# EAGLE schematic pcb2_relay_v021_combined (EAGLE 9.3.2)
Switching done with 23 x G6K-2F-Y 2xDPDT relays + 3 x HC-595

## Sheet 1 of 5: Voltage Controlled Bandpass Filters
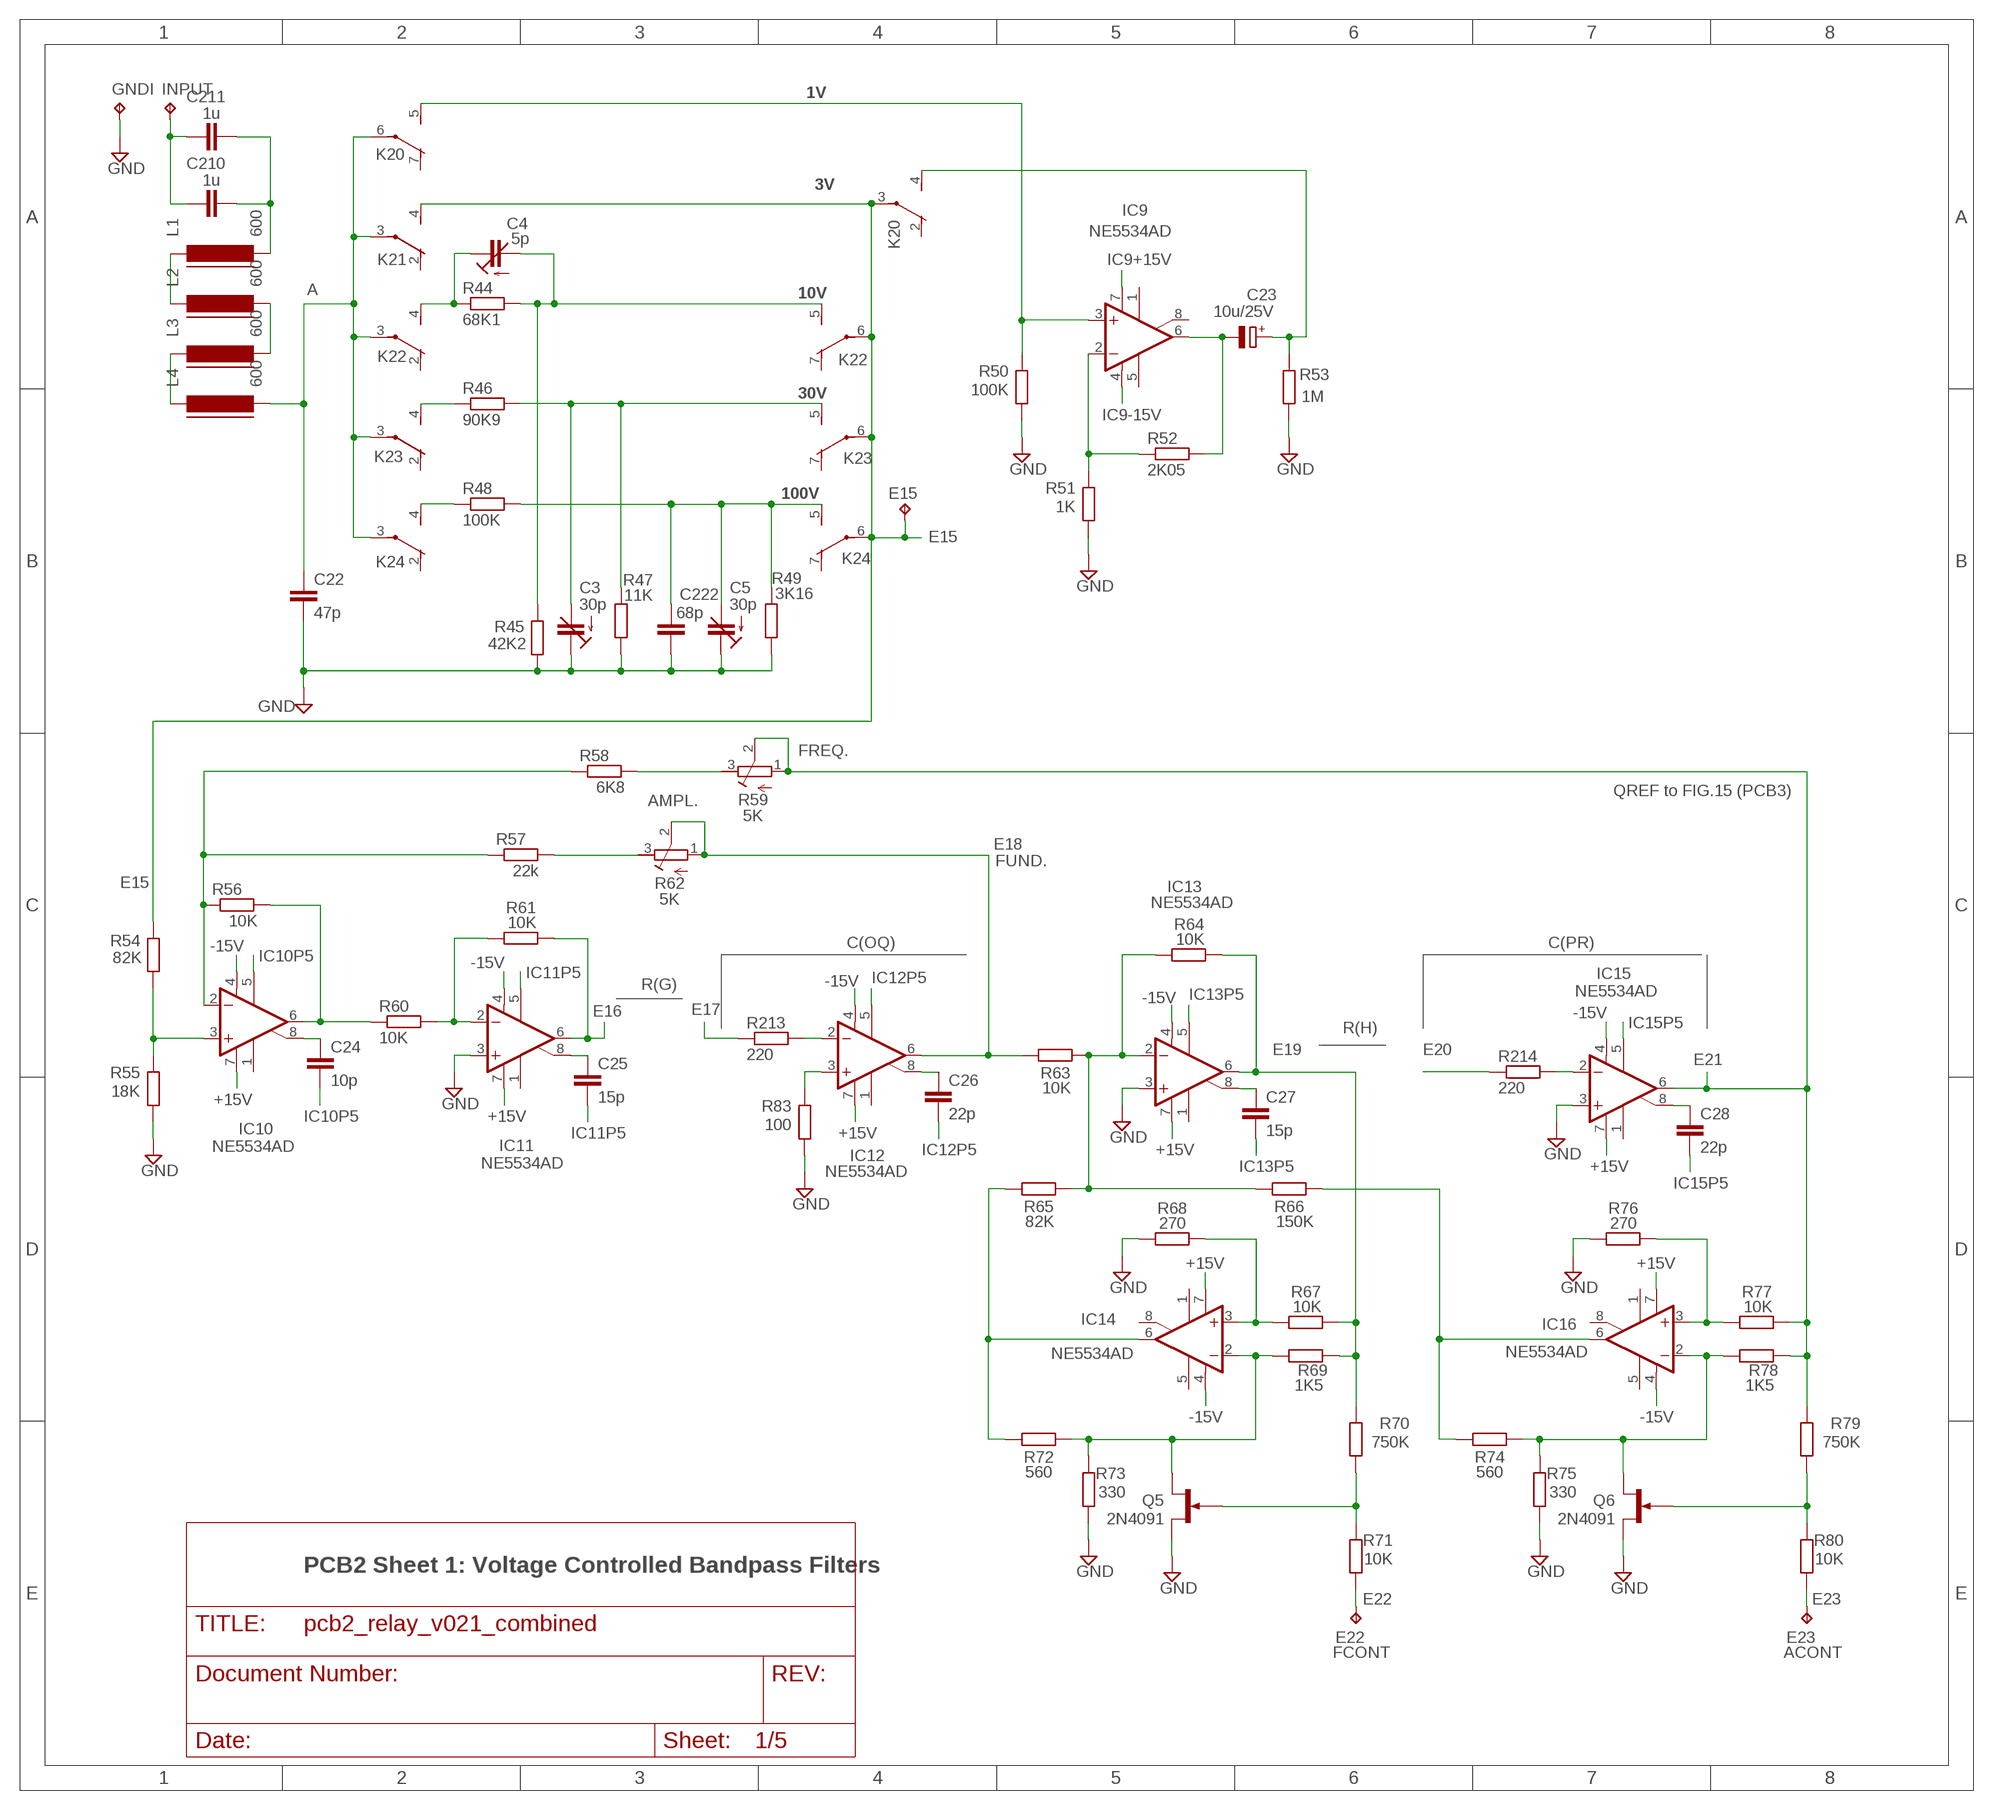
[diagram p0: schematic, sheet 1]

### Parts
C3  30p  C-TRIMM3050.504  [CTRIM3050.504]
C4  5p  C-TRIMM3050.504  [CTRIM3050.504]
C5  30p  C-TRIMM3050.504  [CTRIM3050.504]
C22  47p  C-EU075-042X103  [C075-042X103]
C23  10u/25V  CPOL-EUUD-4X5,8  [UD-4X5,8_NICHICON]
C24  10p  C-EU075-042X103  [C075-042X103]
C25  15p  C-EU075-042X103  [C075-042X103]
C26  22p  C-EU075-042X103  [C075-042X103]
C27  15p  C-EU075-042X103  [C075-042X103]
C28  22p  C-EU075-042X103  [C075-042X103]
C210  1u  C-EU150-072X183  [C150-072X183]
C211  1u  C-EU150-072X183  [C150-072X183]
C222  68p  C-EU075-052X106  [C075-052X106]
E15  TPPAD1-13Y  [P1-13Y]
E22  TPPAD1-13Y  [P1-13Y]
E23  TPPAD1-13Y  [P1-13Y]
GNDI  TPPAD1-13Y  [P1-13Y]
IC9  NE5534AD  [SO08]
IC10  NE5534AD  [SO08]
IC11  NE5534AD  [SO08]
IC12  NE5534AD  [SO08]
IC13  NE5534AD  [SO08]
IC14  NE5534AD  [SO08]
IC15  NE5534AD  [SO08]
IC16  NE5534AD  [SO08]
INPUT  TPPAD1-13Y  [P1-13Y]
K20  G6K-2F-Y  [G6K-2F-Y]
K21  G6K-2F-Y  [G6K-2F-Y]
K22  G6K-2F-Y  [G6K-2F-Y]
K23  G6K-2F-Y  [G6K-2F-Y]
K24  G6K-2F-Y  [G6K-2F-Y]
L1  600  FERRITE-1206  [FB1206]
L2  600  FERRITE-1206  [FB1206]
L3  600  FERRITE-1206  [FB1206]
L4  600  FERRITE-1206  [FB1206]
Q5  2N4091  2N5638  [TO92G]
Q6  2N4091  2N5638  [TO92G]
R44  68K1  R-EU_R1206  [R1206]
R45  42K2  R-EU_R1206  [R1206]
R46  90K9  R-EU_R1206  [R1206]
R47  11K  R-EU_R1206  [R1206]
R48  100K  R-EU_R1206  [R1206]
R49  3K16  R-EU_R1206  [R1206]
R50  100K  R-EU_R1206  [R1206]
R51  1K  R-EU_R1206  [R1206]
R52  2K05  R-EU_R1206  [R1206]
R53  1M  R-EU_R1206  [R1206]
R54  82K  R-EU_R1206  [R1206]
R55  18K  R-EU_R1206  [R1206]
R56  10K  R-EU_R1206  [R1206]
R57  22k  R-EU_R1206  [R1206]
R58  6K8  R-EU_R1206  [R1206]
R59  5K  R-TRIMM3296W  [RTRIM3296W]
R60  10K  R-EU_R1206  [R1206]
R61  10K  R-EU_R1206  [R1206]
R62  5K  R-TRIMM3296W  [RTRIM3296W]
R63  10K  R-EU_R1206  [R1206]
R64  10K  R-EU_R1206  [R1206]
R65  82K  R-EU_R1206  [R1206]
R66  150K  R-EU_R1206  [R1206]
R67  10K  R-EU_R1206  [R1206]
R68  270  R-EU_R1206  [R1206]
R69  1K5  R-EU_R1206  [R1206]
R70  750K  R-EU_R1206  [R1206]
R71  10K  R-EU_R1206  [R1206]
R72  560  R-EU_R1206  [R1206]
R73  330  R-EU_R1206  [R1206]
R74  560  R-EU_R1206  [R1206]
R75  330  R-EU_R1206  [R1206]
R76  270  R-EU_R1206  [R1206]
R77  10K  R-EU_R1206  [R1206]
R78  1K5  R-EU_R1206  [R1206]
R79  750K  R-EU_R1206  [R1206]
R80  10K  R-EU_R1206  [R1206]
R83  100  R-EU_R1206  [R1206]
R213  220  R-EU_R1206  [R1206]
R214  220  R-EU_R1206  [R1206]

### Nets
+15V: IC10.7(V+) IC11.7(V+) IC12.7(V+) IC13.7(V+) IC14.7(V+) IC15.7(V+) IC16.7(V+) ; also sheet 2,4,5
-15V: IC10.4(V-) IC11.4(V-) IC12.4(V-) IC13.4(V-) IC14.4(V-) IC15.4(V-) IC16.4(V-) ; also sheet 2,4,5
A: C22.1 K20.6(3:P) K21.3(2:P) K22.3(2:P) K23.3(2:P) K24.3(2:P) L4.2
E12: IC9.3(+IN) K20.5(3:S) R50.2
E13: C23.+ K20.4(2:S) R53.2
E15: E15.TP K20.3(2:P) K21.4(2:S) K22.6(3:P) K23.6(3:P) K24.6(3:P) R54.2 ; also sheet 2
E16: IC11.6(OUT) R61.2 ; also sheet 3
E17: R213.1 ; also sheet 3
E18: IC12.6(OUT) R62.1(A) R62.2(S) R63.2 ; also sheet 2,3,5
E19: IC13.6(OUT) R64.2 R67.2 R69.2 R70.2 ; also sheet 3
E20: R214.1 ; also sheet 3
E21: IC15.6(OUT) R59.1(A) R59.2(S) R77.2 R78.2 R79.2 ; also sheet 3
E22: E22.TP R71.1 ; also sheet 3
E23: E23.TP R80.1 ; also sheet 3
GND: C3.1(E) C5.1(E) C22.2 C222.2 GNDI.TP IC11.3(+IN) IC13.3(+IN) IC15.3(+IN) Q5.S Q6.S R45.1 R47.1 R49.1 R50.1 R51.1 R53.1 R55.1 R68.1 R73.1 R75.1 R76.1 R83.1 ; also sheet 2,3,4,5
IC9+15V: IC9.7(V+) ; also sheet 4
IC9-15V: IC9.4(V-) ; also sheet 4
IC10P5: C24.2 IC10.5(CMP)
IC11P5: C25.2 IC11.5(CMP)
IC12P5: C26.2 IC12.5(CMP)
IC13P5: C27.2 IC13.5(CMP)
IC15P5: C28.2 IC15.5(CMP)
IN: C210.1 C211.1 INPUT.TP
N$12: C24.1 IC10.8(ON/CMP)
N$26: IC10.6(OUT) R56.2 R60.1
N$27: IC11.2(-IN) R60.2 R61.1
N$31: C25.1 IC11.8(ON/CMP)
N$32: IC12.2(-IN) R213.2
N$33: C23.- IC9.6(OUT) R52.2
N$34: IC9.2(-IN) R51.2 R52.1
N$35: C26.1 IC12.8(ON/CMP)
N$38: IC10.3(+IN) R54.1 R55.2
N$39: IC12.3(+IN) R83.2
N$40: IC13.2(-IN) R63.1 R64.1 R65.1 R66.2
N$41: C27.1 IC13.8(ON/CMP)
N$42: IC14.6(OUT) R65.2 R72.2
N$43: IC14.3(+IN) R67.1 R68.2
N$44: Q5.G R70.1 R71.2
N$45: IC14.2(-IN) Q5.D R69.1 R72.1 R73.2
N$46: IC16.3(+IN) R76.2 R77.1
N$47: Q6.G R79.1 R80.2
N$48: IC16.2(-IN) Q6.D R74.1 R75.2 R78.1
N$49: IC16.6(OUT) R66.1 R74.2
N$51: C28.1 IC15.8(ON/CMP)
N$52: IC15.2(-IN) R214.2
N$53: R57.2 R62.3(E)
N$54: R58.2 R59.3(E)
N$56: IC10.2(-IN) R56.1 R57.1 R58.1
N$119: C210.2 C211.2 L1.2
N$120: C4.2(A) K22.5(3:S) R44.2 R45.2
N$121: L1.1 L2.1
N$122: L2.2 L3.2
N$123: L3.1 L4.1
N$124: C4.1(E) K22.4(2:S) R44.1
N$126: K23.4(2:S) R46.1
N$133: K24.4(2:S) R48.1
N$134: C3.2(A) K23.5(3:S) R46.2 R47.2
N$137: C5.2(A) C222.1 K24.5(3:S) R48.2 R49.2
Unconnected: IC9.1(ON) IC9.5(CMP) IC9.8(ON/CMP) IC10.1(ON) IC11.1(ON) IC12.1(ON) IC13.1(ON) IC14.1(ON) IC14.5(CMP) IC14.8(ON/CMP) IC15.1(ON) IC16.1(ON) IC16.5(CMP) IC16.8(ON/CMP) K20.2(2:O) K20.7(3:O) K21.2(2:O) K22.2(2:O) K22.7(3:O) K23.2(2:O) K23.7(3:O) K24.2(2:O) K24.7(3:O)

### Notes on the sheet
- 1V
- 3V
- 10V
- 30V
- 100V
- FREQ.
- QREF to FIG.15 (PCB3)
- AMPL.
- FUND.
- C(OQ) | C(PR)
- R(G)
- R(H)
- PCB2 Sheet 1: Voltage Controlled Bandpass Filters
- FCONT | ACONT

## Sheet 2 of 5: Product Amplifier and Level Set
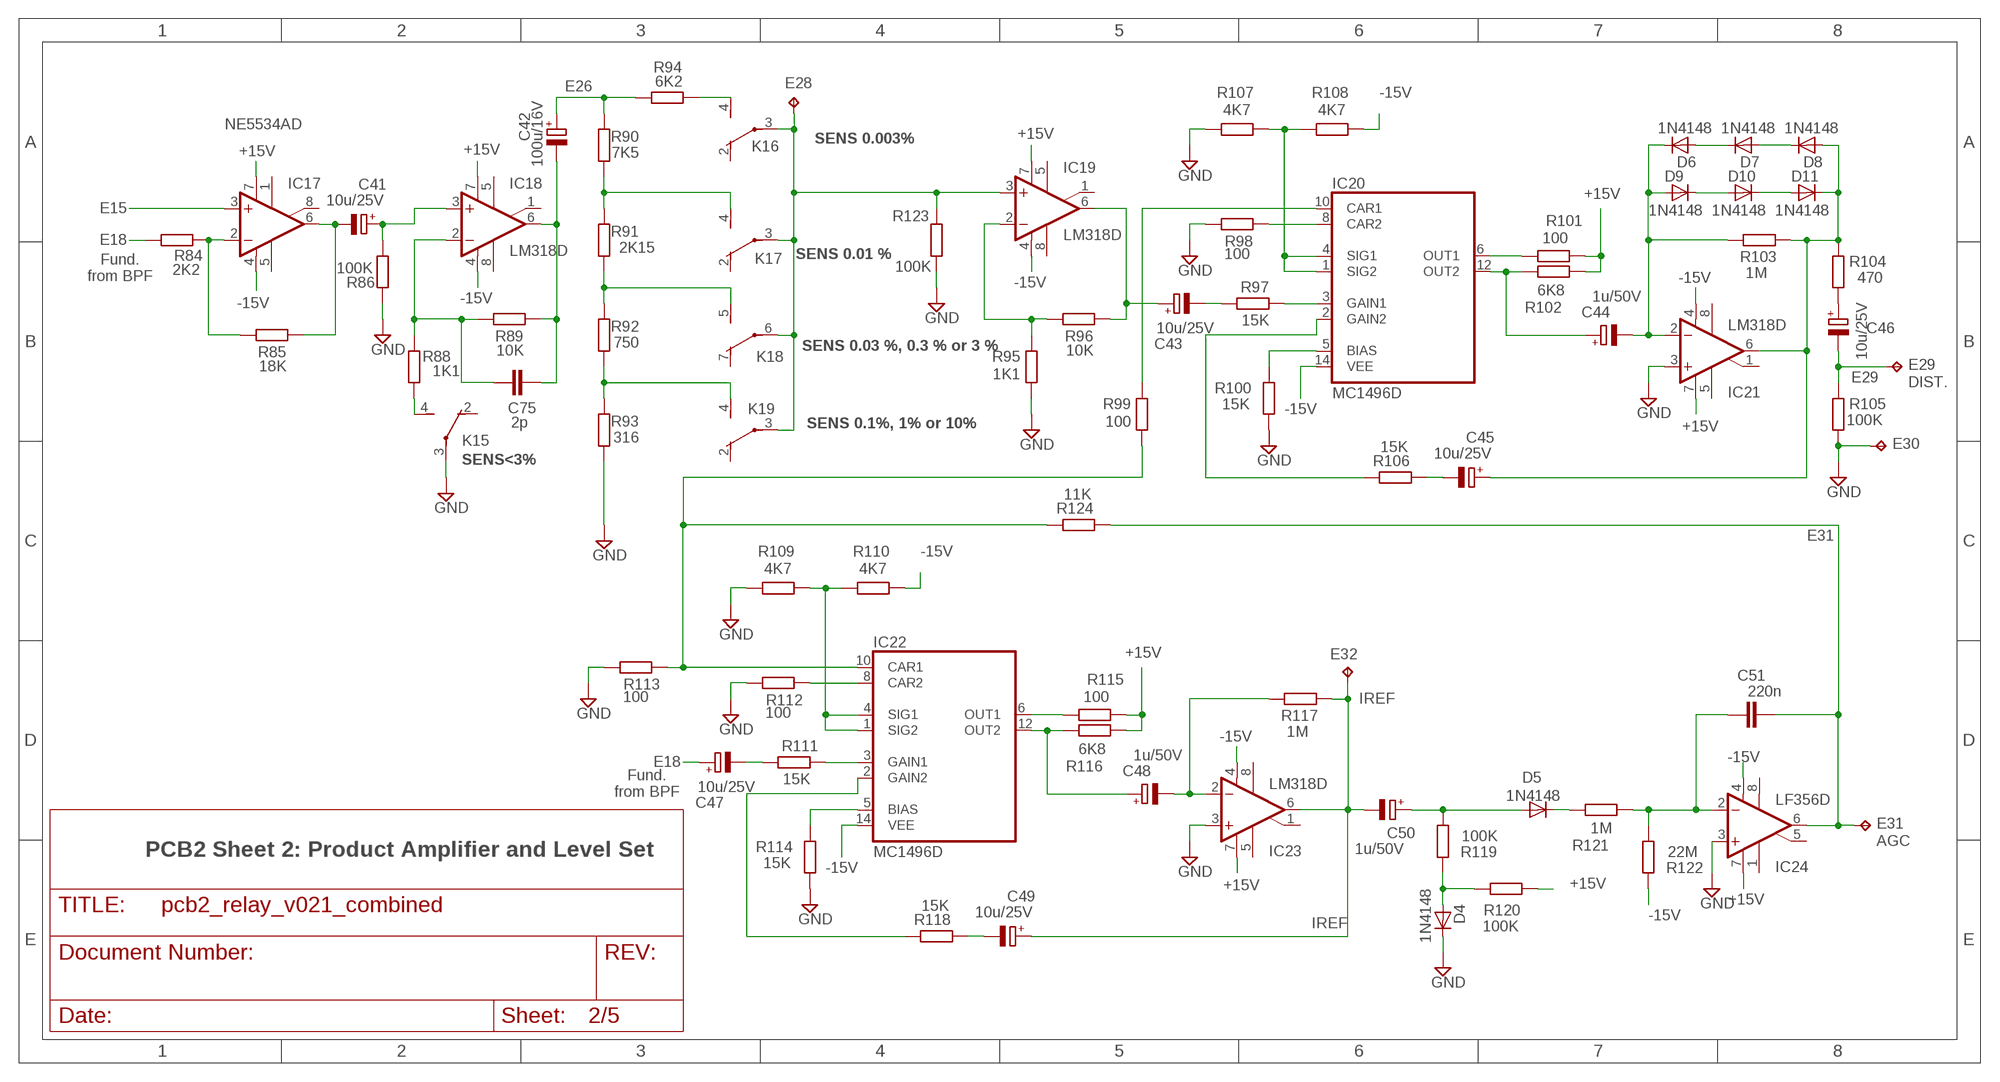
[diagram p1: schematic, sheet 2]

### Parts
C41  10u/25V  CPOL-EUUD-4X5,8  [UD-4X5,8_NICHICON]
C42  100u/16V  CPOL-EUUD-6,3X8,8  [UD-6,3X5,8_NICHICON]
C43  10u/25V  CPOL-EUUD-4X5,8  [UD-4X5,8_NICHICON]
C44  1u/50V  CPOL-EUUD-4X5,8  [UD-4X5,8_NICHICON]
C45  10u/25V  CPOL-EUUD-4X5,8  [UD-4X5,8_NICHICON]
C46  10u/25V  CPOL-EUUD-4X5,8  [UD-4X5,8_NICHICON]
C47  10u/25V  CPOL-EUUD-4X5,8  [UD-4X5,8_NICHICON]
C48  1u/50V  CPOL-EUUD-4X5,8  [UD-4X5,8_NICHICON]
C49  10u/25V  CPOL-EUUD-4X5,8  [UD-4X5,8_NICHICON]
C50  1u/50V  CPOL-EUUD-4X5,8  [UD-4X5,8_NICHICON]
C51  220n  C-EU075-052X106  [C075-052X106]
C75  2p  C-EUC1206  [C1206]
D4  1N4148  D-SOD-80  [SOD80]
D5  1N4148  D-SOD-80  [SOD80]
D6  1N4148  D-SOD-80  [SOD80]
D7  1N4148  D-SOD-80  [SOD80]
D8  1N4148  D-SOD-80  [SOD80]
D9  1N4148  D-SOD-80  [SOD80]
D10  1N4148  D-SOD-80  [SOD80]
D11  1N4148  D-SOD-80  [SOD80]
E28  TPPAD1-13Y  [P1-13Y]
E29  TPPAD1-13Y  [P1-13Y]
E30  TPPAD1-13Y  [P1-13Y]
E31  TPPAD1-13Y  [P1-13Y]
E32  TPPAD1-13Y  [P1-13Y]
IC17  NE5534AD  [SO08]
IC18  LM318D  [SO08]
IC19  LM318D  [SO08]
IC20  MC1496D  [SOIC-14]
IC21  LM318D  [SO08]
IC22  MC1496D  [SOIC-14]
IC23  LM318D  [SO08]
IC24  LF356D  [SO08]
K15  G6K-2F-Y  [G6K-2F-Y]
K16  G6K-2F-Y  [G6K-2F-Y]
K17  G6K-2F-Y  [G6K-2F-Y]
K18  G6K-2F-Y  [G6K-2F-Y]
K19  G6K-2F-Y  [G6K-2F-Y]
R84  2K2  R-EU_R1206  [R1206]
R85  18K  R-EU_R1206  [R1206]
R86  100K  R-EU_R1206  [R1206]
R88  1K1  R-EU_R1206  [R1206]
R89  10K  R-EU_R1206  [R1206]
R90  7K5  R-EU_R1206  [R1206]
R91  2K15  R-EU_R1206  [R1206]
R92  750  R-EU_R1206  [R1206]
R93  316  R-EU_R1206  [R1206]
R94  6K2  R-EU_R1206  [R1206]
R95  1K1  R-EU_R1206  [R1206]
R96  10K  R-EU_R1206  [R1206]
R97  15K  R-EU_R1206  [R1206]
R98  100  R-EU_R1206  [R1206]
R99  100  R-EU_R1206  [R1206]
R100  15K  R-EU_R1206  [R1206]
R101  100  R-EU_R1206  [R1206]
R102  6K8  R-EU_R1206  [R1206]
R103  1M  R-EU_R1206  [R1206]
R104  470  R-EU_R1206  [R1206]
R105  100K  R-EU_R1206  [R1206]
R106  15K  R-EU_R1206  [R1206]
R107  4K7  R-EU_R1206  [R1206]
R108  4K7  R-EU_R1206  [R1206]
R109  4K7  R-EU_R1206  [R1206]
R110  4K7  R-EU_R1206  [R1206]
R111  15K  R-EU_R1206  [R1206]
R112  100  R-EU_R1206  [R1206]
R113  100  R-EU_R1206  [R1206]
R114  15K  R-EU_R1206  [R1206]
R115  100  R-EU_R1206  [R1206]
R116  6K8  R-EU_R1206  [R1206]
R117  1M  R-EU_R1206  [R1206]
R118  15K  R-EU_R1206  [R1206]
R119  100K  R-EU_R1206  [R1206]
R120  100K  R-EU_R1206  [R1206]
R121  1M  R-EU_R1206  [R1206]
R122  22M  R-EU_R1206  [R1206]
R123  100K  R-EU_R1206  [R1206]
R124  11K  R-EU_R1206  [R1206]

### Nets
+15V: IC17.7(V+) IC18.7(V+) IC19.7(V+) IC21.7(V+) IC23.7(V+) IC24.7(V+) R101.1 R102.2 R115.1 R116.2 R120.1 ; also sheet 1,4,5
-15V: IC17.4(V-) IC18.4(V-) IC19.4(V-) IC20.14(VEE) IC21.4(V-) IC22.14(VEE) IC23.4(V-) IC24.4(V-) R108.2 R110.2 R122.1 ; also sheet 1,4,5
E15: IC17.3(+IN) ; also sheet 1
E18: C47.+ R84.2 ; also sheet 1,3,5
E25: K15.4(2:S) R88.2
E26: C42.+ R90.1 R94.2
E28: E28.TP IC19.3(+IN) K16.3(2:P) K17.3(2:P) K18.6(3:P) K19.3(2:P) R123.2
E29: C46.- E29.TP R105.1 ; also sheet 3
E31: C51.2 E31.TP IC24.6(OUT) R124.2 ; also sheet 3
GND: D4.1(C) E30.TP IC21.3(+IN) IC23.3(+IN) IC24.3(+IN) K15.3(2:P) R86.1 R93.2 R95.2 R98.2 R100.2 R105.2 R107.1 R109.1 R112.2 R113.2 R114.2 R123.1 ; also sheet 1,3,4,5
IREF: C49.+ C50.- E32.TP IC23.6(OUT) R117.2 ; also sheet 3
N$3: K19.4(2:S) R92.2 R93.1
N$4: K18.5(3:S) R91.2 R92.1
N$5: K17.4(2:S) R90.2 R91.1
N$6: K16.4(2:S) R94.1
N$17: IC17.2(-IN) R84.1 R85.2
N$22: C41.- IC17.6(OUT) R85.1
N$24: C41.+ IC18.3(+IN) R86.2
N$28: C75.2 IC18.2(-IN) R88.1 R89.2
N$29: C42.- C75.1 IC18.6(OUT) R89.1
N$36: IC19.2(-IN) R95.1 R96.2
N$37: C43.+ IC19.6(OUT) R96.1
N$57: C43.- R97.2
N$58: IC20.3(GAIN1) R97.1
N$59: IC20.5(BIAS) R100.1
N$60: IC20.2(GAIN2) R106.1
N$61: C45.- R106.2
N$62: IC20.1(SIG2) IC20.4(SIG1) R107.2 R108.1
N$64: IC20.8(CAR2) R98.1
N$65: IC20.10(CAR1) R99.1
N$66: IC20.6(OUT1) R101.2
N$67: C44.+ IC20.12(OUT2) R102.1
N$68: C45.+ D8.2(A) D11.1(C) IC21.6(OUT) R103.2 R104.1
N$69: C44.- D6.1(C) D9.2(A) IC21.2(-IN) R103.1
N$70: D9.1(C) D10.2(A)
N$125: D10.1(C) D11.2(A)
N$135: D7.2(A) D8.1(C)
N$136: D6.2(A) D7.1(C)
N$138: C46.+ R104.2
N$139: C47.- R111.2
N$157: IC22.3(GAIN1) R111.1
N$158: IC22.5(BIAS) R114.1
N$159: IC22.2(GAIN2) R118.1
N$160: C49.- R118.2
N$161: IC22.1(SIG2) IC22.4(SIG1) R109.2 R110.1
N$162: IC22.8(CAR2) R112.1
N$163: IC22.6(OUT1) R115.2
N$164: C48.+ IC22.12(OUT2) R116.1
N$165: C48.- IC23.2(-IN) R117.1
N$166: IC22.10(CAR1) R99.2 R113.1 R124.1
N$167: C51.1 IC24.2(-IN) R121.2 R122.2
N$168: D5.1(C) R121.1
N$169: D4.2(A) R119.1 R120.2
N$170: C50.+ D5.2(A) R119.2
Unconnected: IC17.1(ON) IC17.5(CMP) IC17.8(ON/CMP) IC18.1(ON/CMP) IC18.5(ON) IC18.8(CMP) IC19.1(ON/CMP) IC19.5(ON) IC19.8(CMP) IC21.1(ON/CMP) IC21.5(ON) IC21.8(CMP) IC23.1(ON/CMP) IC23.5(ON) IC23.8(CMP) IC24.1(ON1) IC24.5(ON2) IC24.8(OPT) K15.2(2:O) K16.2(2:O) K17.2(2:O) K18.7(3:O) K19.2(2:O)

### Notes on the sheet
- SENS 0.003%
- SENS 0.01 %
- Fund.
  from BPF
- SENS 0.03 %, 0.3 % or 3 %
- DIST.
- SENS 0.1%, 1% or 10%
- SENS<3%
- IREF
- Fund.
  from BPF
- AGC
- PCB2 Sheet 2: Product Amplifier and Level Set

## Sheet 3 of 5: Relays + Digital Logic
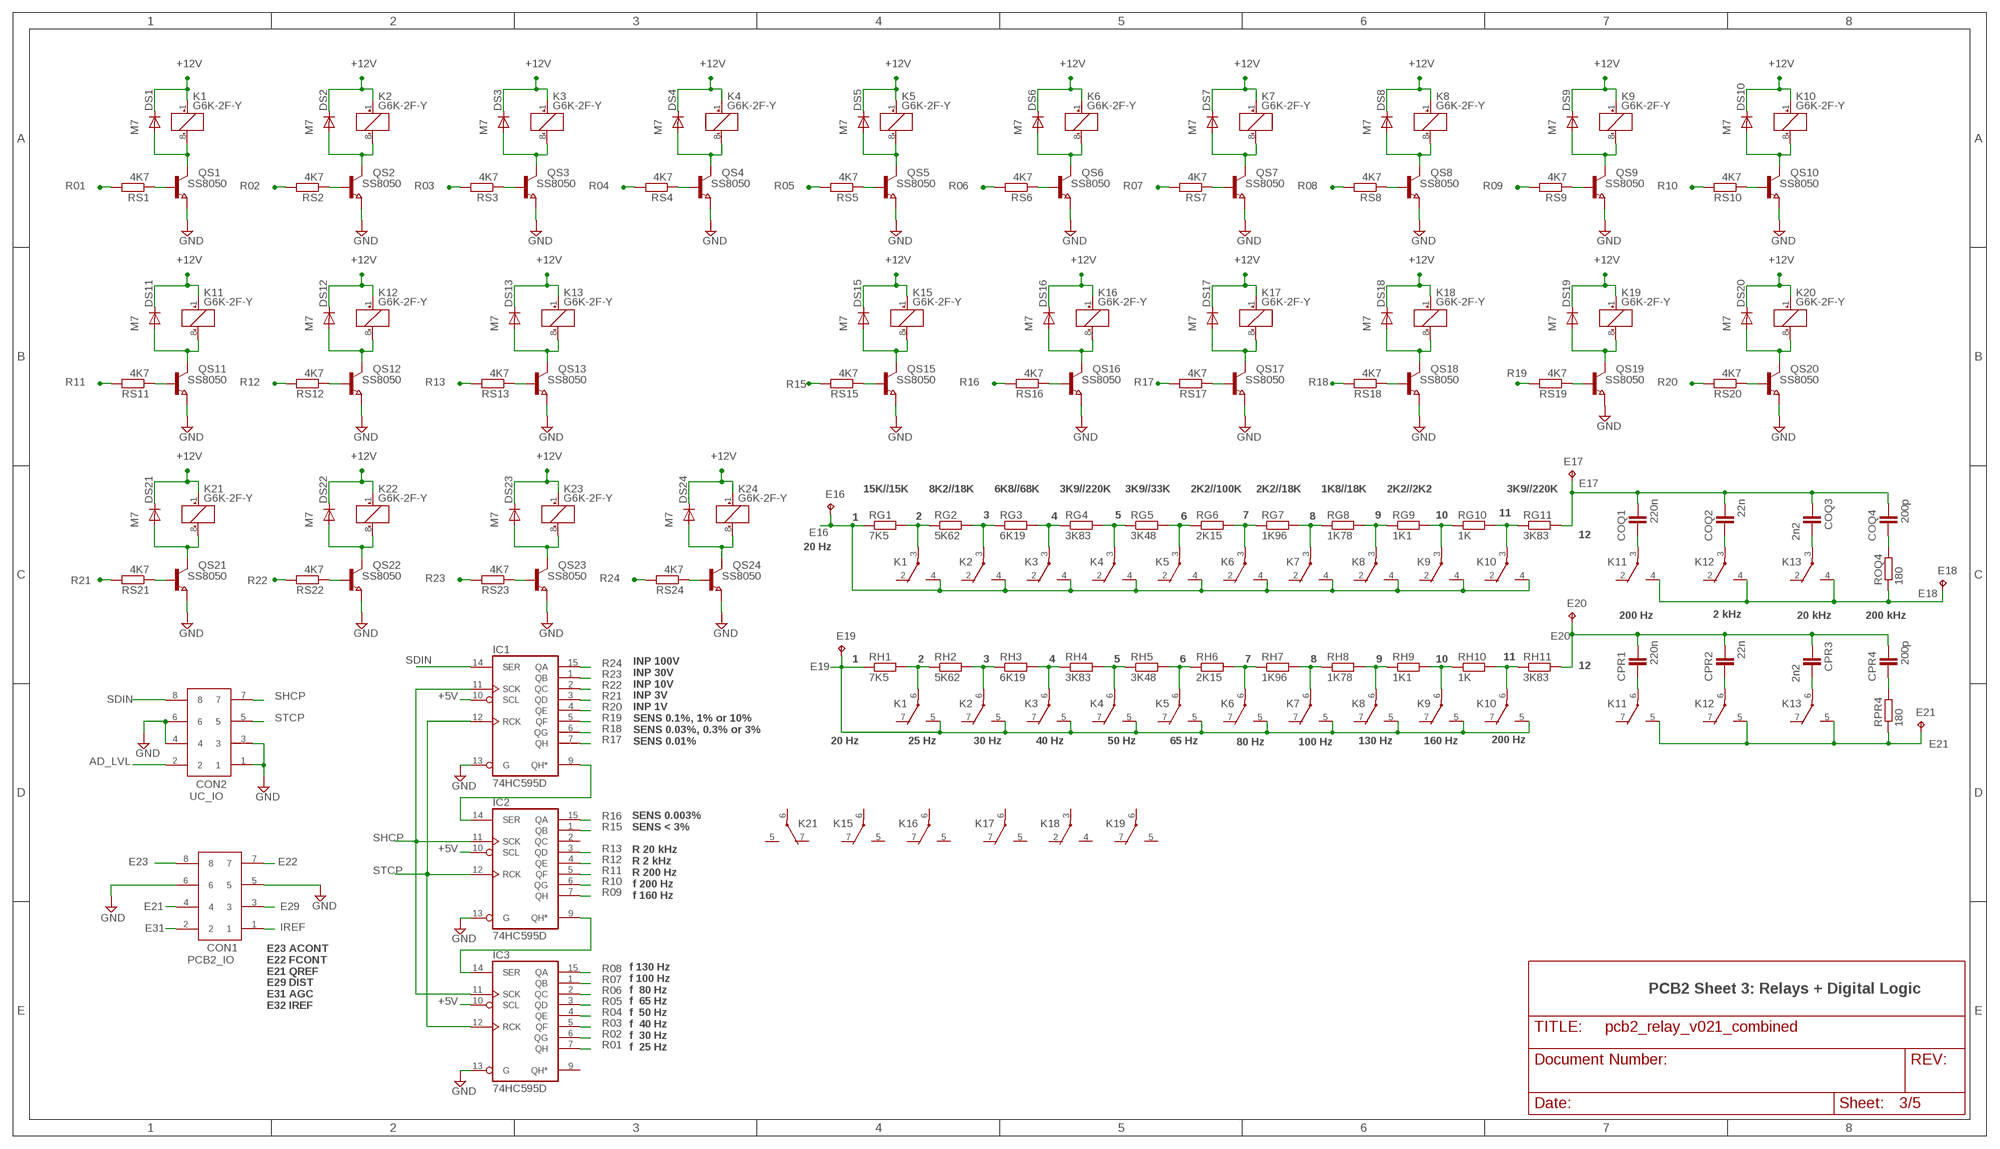
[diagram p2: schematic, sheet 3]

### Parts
CON1  PCB2_IO  61200821621  [61200821621]
CON2  UC_IO  61200821621  [61200821621]
COQ1  220n  C-EU075-052X106  [C075-052X106]
COQ2  22n  C-EU050-045X075  [C050-045X075]
COQ3  2n2  C-EU075-052X106  [C075-052X106]
COQ4  200p  C-EU102-043X133  [C102-043X133]
CPR1  220n  C-EU075-052X106  [C075-052X106]
CPR2  22n  C-EU050-045X075  [C050-045X075]
CPR3  2n2  C-EU075-052X106  [C075-052X106]
CPR4  200p  C-EU102-043X133  [C102-043X133]
DS1  M7  DIODE-DO214AC  [DO214AC]
DS2  M7  DIODE-DO214AC  [DO214AC]
DS3  M7  DIODE-DO214AC  [DO214AC]
DS4  M7  DIODE-DO214AC  [DO214AC]
DS5  M7  DIODE-DO214AC  [DO214AC]
DS6  M7  DIODE-DO214AC  [DO214AC]
DS7  M7  DIODE-DO214AC  [DO214AC]
DS8  M7  DIODE-DO214AC  [DO214AC]
DS9  M7  DIODE-DO214AC  [DO214AC]
DS10  M7  DIODE-DO214AC  [DO214AC]
DS11  M7  DIODE-DO214AC  [DO214AC]
DS12  M7  DIODE-DO214AC  [DO214AC]
DS13  M7  DIODE-DO214AC  [DO214AC]
DS15  M7  DIODE-DO214AC  [DO214AC]
DS16  M7  DIODE-DO214AC  [DO214AC]
DS17  M7  DIODE-DO214AC  [DO214AC]
DS18  M7  DIODE-DO214AC  [DO214AC]
DS19  M7  DIODE-DO214AC  [DO214AC]
DS20  M7  DIODE-DO214AC  [DO214AC]
DS21  M7  DIODE-DO214AC  [DO214AC]
DS22  M7  DIODE-DO214AC  [DO214AC]
DS23  M7  DIODE-DO214AC  [DO214AC]
DS24  M7  DIODE-DO214AC  [DO214AC]
E16  TPPAD1-13Y  [P1-13Y]
E17  TPPAD1-13Y  [P1-13Y]
E18  TPPAD1-13Y  [P1-13Y]
E19  TPPAD1-13Y  [P1-13Y]
E20  TPPAD1-13Y  [P1-13Y]
E21  TPPAD1-13Y  [P1-13Y]
IC1  74HC595D  [SO16]
IC2  74HC595D  [SO16]
IC3  74HC595D  [SO16]
K1  G6K-2F-Y  [G6K-2F-Y]
K2  G6K-2F-Y  [G6K-2F-Y]
K3  G6K-2F-Y  [G6K-2F-Y]
K4  G6K-2F-Y  [G6K-2F-Y]
K5  G6K-2F-Y  [G6K-2F-Y]
K6  G6K-2F-Y  [G6K-2F-Y]
K7  G6K-2F-Y  [G6K-2F-Y]
K8  G6K-2F-Y  [G6K-2F-Y]
K9  G6K-2F-Y  [G6K-2F-Y]
K10  G6K-2F-Y  [G6K-2F-Y]
K11  G6K-2F-Y  [G6K-2F-Y]
K12  G6K-2F-Y  [G6K-2F-Y]
K13  G6K-2F-Y  [G6K-2F-Y]
QS1  SS8050  NPN-TRANSISTOR_SOT23  [SOT23]
QS2  SS8050  NPN-TRANSISTOR_SOT23  [SOT23]
QS3  SS8050  NPN-TRANSISTOR_SOT23  [SOT23]
QS4  SS8050  NPN-TRANSISTOR_SOT23  [SOT23]
QS5  SS8050  NPN-TRANSISTOR_SOT23  [SOT23]
QS6  SS8050  NPN-TRANSISTOR_SOT23  [SOT23]
QS7  SS8050  NPN-TRANSISTOR_SOT23  [SOT23]
QS8  SS8050  NPN-TRANSISTOR_SOT23  [SOT23]
QS9  SS8050  NPN-TRANSISTOR_SOT23  [SOT23]
QS10  SS8050  NPN-TRANSISTOR_SOT23  [SOT23]
QS11  SS8050  NPN-TRANSISTOR_SOT23  [SOT23]
QS12  SS8050  NPN-TRANSISTOR_SOT23  [SOT23]
QS13  SS8050  NPN-TRANSISTOR_SOT23  [SOT23]
QS15  SS8050  NPN-TRANSISTOR_SOT23  [SOT23]
QS16  SS8050  NPN-TRANSISTOR_SOT23  [SOT23]
QS17  SS8050  NPN-TRANSISTOR_SOT23  [SOT23]
QS18  SS8050  NPN-TRANSISTOR_SOT23  [SOT23]
QS19  SS8050  NPN-TRANSISTOR_SOT23  [SOT23]
QS20  SS8050  NPN-TRANSISTOR_SOT23  [SOT23]
QS21  SS8050  NPN-TRANSISTOR_SOT23  [SOT23]
QS22  SS8050  NPN-TRANSISTOR_SOT23  [SOT23]
QS23  SS8050  NPN-TRANSISTOR_SOT23  [SOT23]
QS24  SS8050  NPN-TRANSISTOR_SOT23  [SOT23]
RG1  7K5  R-EU_R1206  [R1206]
RG2  5K62  R-EU_R1206  [R1206]
RG3  6K19  R-EU_R1206  [R1206]
RG4  3K83  R-EU_R1206  [R1206]
RG5  3K48  R-EU_R1206  [R1206]
RG6  2K15  R-EU_R1206  [R1206]
RG7  1K96  R-EU_R1206  [R1206]
RG8  1K78  R-EU_R1206  [R1206]
RG9  1K1  R-EU_R1206  [R1206]
RG10  1K  R-EU_R1206  [R1206]
RG11  3K83  R-EU_R1206  [R1206]
RH1  7K5  R-EU_R1206  [R1206]
RH2  5K62  R-EU_R1206  [R1206]
RH3  6K19  R-EU_R1206  [R1206]
RH4  3K83  R-EU_R1206  [R1206]
RH5  3K48  R-EU_R1206  [R1206]
RH6  2K15  R-EU_R1206  [R1206]
RH7  1K96  R-EU_R1206  [R1206]
RH8  1K78  R-EU_R1206  [R1206]
RH9  1K1  R-EU_R1206  [R1206]
RH10  1K  R-EU_R1206  [R1206]
RH11  3K83  R-EU_R1206  [R1206]
ROQ4  180  R-EU_R1206  [R1206]
RPR4  180  R-EU_R1206  [R1206]
RS1  4K7  R-EU_R1206  [R1206]
RS2  4K7  R-EU_R1206  [R1206]
RS3  4K7  R-EU_R1206  [R1206]
RS4  4K7  R-EU_R1206  [R1206]
RS5  4K7  R-EU_R1206  [R1206]
RS6  4K7  R-EU_R1206  [R1206]
RS7  4K7  R-EU_R1206  [R1206]
RS8  4K7  R-EU_R1206  [R1206]
RS9  4K7  R-EU_R1206  [R1206]
RS10  4K7  R-EU_R1206  [R1206]
RS11  4K7  R-EU_R1206  [R1206]
RS12  4K7  R-EU_R1206  [R1206]
RS13  4K7  R-EU_R1206  [R1206]
RS15  4K7  R-EU_R1206  [R1206]
RS16  4K7  R-EU_R1206  [R1206]
RS17  4K7  R-EU_R1206  [R1206]
RS18  4K7  R-EU_R1206  [R1206]
RS19  4K7  R-EU_R1206  [R1206]
RS20  4K7  R-EU_R1206  [R1206]
RS21  4K7  R-EU_R1206  [R1206]
RS22  4K7  R-EU_R1206  [R1206]
RS23  4K7  R-EU_R1206  [R1206]
RS24  4K7  R-EU_R1206  [R1206]

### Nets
+5V: IC1.10(SCL) IC2.10(SCL) IC3.10(SCL) ; also sheet 4
+12V: DS1.C DS2.C DS3.C DS4.C DS5.C DS6.C DS7.C DS8.C DS9.C DS10.C DS11.C DS12.C DS13.C DS15.C DS16.C DS17.C DS18.C DS19.C DS20.C DS21.C DS22.C DS23.C DS24.C K1.1(1:+) K2.1(1:+) K3.1(1:+) K4.1(1:+) K5.1(1:+) K6.1(1:+) K7.1(1:+) K8.1(1:+) K9.1(1:+) K10.1(1:+) K11.1(1:+) K12.1(1:+) K13.1(1:+) K15.1(1:+) K16.1(1:+) K17.1(1:+) K18.1(1:+) K19.1(1:+) K20.1(1:+) K21.1(1:+) K22.1(1:+) K23.1(1:+) K24.1(1:+) ; also sheet 4
AD_LVL: CON2.2 ; also sheet 5
E16: E16.TP K1.4(2:S) K2.4(2:S) K3.4(2:S) K4.4(2:S) K5.4(2:S) K6.4(2:S) K7.4(2:S) K8.4(2:S) K9.4(2:S) K10.4(2:S) RG1.1 ; also sheet 1
E17: COQ1.2 COQ2.2 COQ3.1 COQ4.2 E17.TP RG11.2 ; also sheet 1
E18: E18.TP K11.4(2:S) K12.4(2:S) K13.4(2:S) ROQ4.1 ; also sheet 1,2,5
E19: E19.TP K1.5(3:S) K2.5(3:S) K3.5(3:S) K4.5(3:S) K5.5(3:S) K6.5(3:S) K7.5(3:S) K8.5(3:S) K9.5(3:S) K10.5(3:S) RH1.1 ; also sheet 1
E20: CPR1.2 CPR2.2 CPR3.1 CPR4.2 E20.TP RH11.2 ; also sheet 1
E21: CON1.4 E21.TP K11.5(3:S) K12.5(3:S) K13.5(3:S) RPR4.1 ; also sheet 1
E22: CON1.7 ; also sheet 1
E23: CON1.8 ; also sheet 1
E29: CON1.3 ; also sheet 2
E31: CON1.2 ; also sheet 2
GND: CON1.5 CON1.6 CON2.1 CON2.3 CON2.4 CON2.6 IC1.13(G) IC2.13(G) IC3.13(G) QS1.2(E) QS2.2(E) QS3.2(E) QS4.2(E) QS5.2(E) QS6.2(E) QS7.2(E) QS8.2(E) QS9.2(E) QS10.2(E) QS11.2(E) QS12.2(E) QS13.2(E) QS15.2(E) QS16.2(E) QS17.2(E) QS18.2(E) QS19.2(E) QS20.2(E) QS21.2(E) QS22.2(E) QS23.2(E) QS24.2(E) ; also sheet 1,2,4,5
IREF: CON1.1 ; also sheet 2
N$7: QS19.1(B) RS19.1
N$8: DS19.A K19.8(1:-) QS19.3(C)
N$30: K1.3(2:P) RG1.2 RG2.1
N$55: K2.3(2:P) RG2.2 RG3.1
N$63: K3.3(2:P) RG3.2 RG4.1
N$71: K4.3(2:P) RG4.2 RG5.1
N$72: K5.3(2:P) RG5.2 RG6.1
N$73: K6.3(2:P) RG6.2 RG7.1
N$74: K7.3(2:P) RG7.2 RG8.1
N$75: K8.3(2:P) RG8.2 RG9.1
N$76: K9.3(2:P) RG9.2 RG10.1
N$77: K10.3(2:P) RG10.2 RG11.1
N$78: K1.6(3:P) RH1.2 RH2.1
N$79: K2.6(3:P) RH2.2 RH3.1
N$80: K3.6(3:P) RH3.2 RH4.1
N$81: K4.6(3:P) RH4.2 RH5.1
N$82: K5.6(3:P) RH5.2 RH6.1
N$83: K6.6(3:P) RH6.2 RH7.1
N$84: K7.6(3:P) RH7.2 RH8.1
N$85: K8.6(3:P) RH8.2 RH9.1
N$86: K9.6(3:P) RH9.2 RH10.1
N$87: K10.6(3:P) RH10.2 RH11.1
N$88: QS1.1(B) RS1.1
N$89: DS1.A K1.8(1:-) QS1.3(C)
N$90: QS2.1(B) RS2.1
N$91: DS2.A K2.8(1:-) QS2.3(C)
N$92: QS3.1(B) RS3.1
N$93: DS3.A K3.8(1:-) QS3.3(C)
N$94: QS4.1(B) RS4.1
N$95: DS4.A K4.8(1:-) QS4.3(C)
N$96: QS5.1(B) RS5.1
N$97: DS5.A K5.8(1:-) QS5.3(C)
N$98: QS6.1(B) RS6.1
N$99: DS6.A K6.8(1:-) QS6.3(C)
N$100: QS7.1(B) RS7.1
N$101: DS7.A K7.8(1:-) QS7.3(C)
N$102: QS8.1(B) RS8.1
N$103: DS8.A K8.8(1:-) QS8.3(C)
N$104: QS9.1(B) RS9.1
N$105: DS9.A K9.8(1:-) QS9.3(C)
N$106: QS10.1(B) RS10.1
N$107: DS10.A K10.8(1:-) QS10.3(C)
N$108: COQ1.1 K11.3(2:P)
N$109: COQ2.1 K12.3(2:P)
N$110: COQ3.2 K13.3(2:P)
N$111: QS11.1(B) RS11.1
N$112: DS11.A K11.8(1:-) QS11.3(C)
N$113: QS12.1(B) RS12.1
N$114: DS12.A K12.8(1:-) QS12.3(C)
N$115: QS13.1(B) RS13.1
N$116: DS13.A K13.8(1:-) QS13.3(C)
N$117: QS20.1(B) RS20.1
N$118: DS20.A K20.8(1:-) QS20.3(C)
N$127: QS22.1(B) RS22.1
N$128: DS22.A K22.8(1:-) QS22.3(C)
N$129: QS23.1(B) RS23.1
N$130: DS23.A K23.8(1:-) QS23.3(C)
N$131: QS24.1(B) RS24.1
N$132: DS24.A K24.8(1:-) QS24.3(C)
N$140: QS15.1(B) RS15.1
N$141: DS15.A K15.8(1:-) QS15.3(C)
N$142: QS16.1(B) RS16.1
N$143: DS16.A K16.8(1:-) QS16.3(C)
N$144: QS17.1(B) RS17.1
N$145: DS17.A K17.8(1:-) QS17.3(C)
N$146: QS18.1(B) RS18.1
N$147: DS18.A K18.8(1:-) QS18.3(C)
N$148: QS21.1(B) RS21.1
N$149: DS21.A K21.8(1:-) QS21.3(C)
N$150: IC1.9(QH*) IC2.14(SER)
N$151: IC2.9(QH*) IC3.14(SER)
N$152: CPR1.1 K11.6(3:P)
N$153: CPR2.1 K12.6(3:P)
N$154: CPR3.2 K13.6(3:P)
N$155: COQ4.1 ROQ4.2
N$156: CPR4.1 RPR4.2
R01: IC3.7(QH) RS1.2
R02: IC3.6(QG) RS2.2
R03: IC3.5(QF) RS3.2
R04: IC3.4(QE) RS4.2
R05: IC3.3(QD) RS5.2
R06: IC3.2(QC) RS6.2
R07: IC3.1(QB) RS7.2
R08: IC3.15(QA) RS8.2
R09: IC2.7(QH) RS9.2
R10: IC2.6(QG) RS10.2
R11: IC2.5(QF) RS11.2
R12: IC2.4(QE) RS12.2
R13: IC2.3(QD) RS13.2
R15: IC2.1(QB) RS15.2
R16: IC2.15(QA) RS16.2
R17: IC1.7(QH) RS17.2
R18: IC1.6(QG) RS18.2
R19: IC1.5(QF) RS19.2
R20: IC1.4(QE) RS20.2
R21: IC1.3(QD) RS21.2
R22: IC1.2(QC) RS22.2
R23: IC1.1(QB) RS23.2
R24: IC1.15(QA) RS24.2
SDIN: CON2.8 IC1.14(SER)
SHCP: CON2.7 IC1.11(SCK) IC2.11(SCK) IC3.11(SCK)
STCP: CON2.5 IC1.12(RCK) IC2.12(RCK) IC3.12(RCK)
Unconnected: IC2.2(QC) IC3.9(QH*) K1.2(2:O) K1.7(3:O) K2.2(2:O) K2.7(3:O) K3.2(2:O) K3.7(3:O) K4.2(2:O) K4.7(3:O) K5.2(2:O) K5.7(3:O) K6.2(2:O) K6.7(3:O) K7.2(2:O) K7.7(3:O) K8.2(2:O) K8.7(3:O) K9.2(2:O) K9.7(3:O) K10.2(2:O) K10.7(3:O) K11.2(2:O) K11.7(3:O) K12.2(2:O) K12.7(3:O) K13.2(2:O) K13.7(3:O) K15.5(3:S) K15.6(3:P) K15.7(3:O) K16.5(3:S) K16.6(3:P) K16.7(3:O) K17.5(3:S) K17.6(3:P) K17.7(3:O) K18.2(2:O) K18.3(2:P) K18.4(2:S) K19.5(3:S) K19.6(3:P) K19.7(3:O) K21.5(3:S) K21.6(3:P) K21.7(3:O)

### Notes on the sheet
- 15K//15K | 8K2//18K | 6K8//68K | 3K9//220K | 3K9//33K | 2K2//100K | 2K2//18K | 1K8//18K | 2K2//2K2 | 3K9//220K
- 3 | 5 | 7 | 9 | 10 | 11
- 1 | 2 | 4 | 6 | 8
- 12
- 20 Hz
- 200 Hz | 2 kHz | 20 kHz | 200 kHz
- 1 | 2 | 3 | 4 | 5 | 6 | 7 | 8 | 9 | 10 | 11
- 12
- 20 Hz | 25 Hz | 30 Hz | 40 Hz | 50 Hz | 65 Hz | 80 Hz | 100 Hz | 130 Hz | 160 Hz | 200 Hz
- INP 100V
  INP 30V
  INP 10V
  INP 3V
  INP 1V
  SENS 0.1%, 1% or 10%
  SENS 0.03%, 0.3% or 3%
  SENS 0.01%
- SENS 0.003%
  SENS < 3%
  
  R 20 kHz
  R 2 kHz
  R 200 Hz
  f 200 Hz
  f 160 Hz
- PCB2 Sheet 3: Relays + Digital Logic
- E23 ACONT
  E22 FCONT
  E21 QREF
  E29 DIST
  E31 AGC
  E32 IREF
- f 130 Hz
  f 100 Hz
  f  80 Hz
  f  65 Hz
  f  50 Hz
  f  40 Hz
  f  30 Hz
  f  25 Hz

## Sheet 4 of 5: Power-Supply
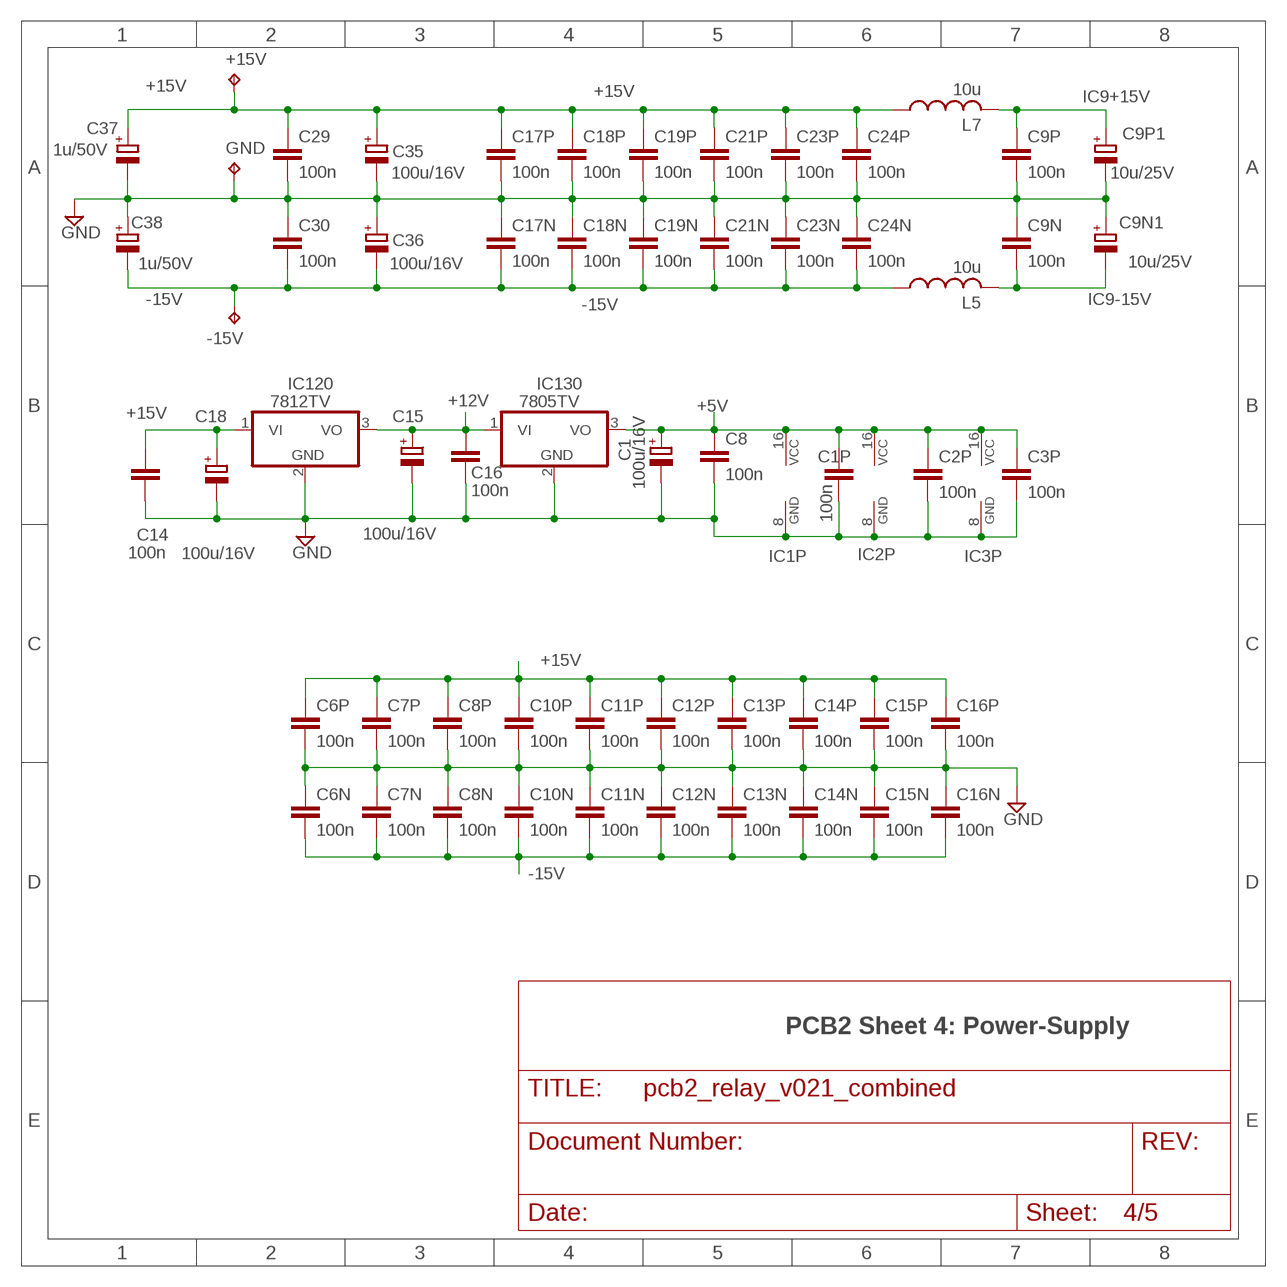
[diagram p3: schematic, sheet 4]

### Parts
+15V  TPPAD1-13Y  [P1-13Y]
-15V  TPPAD1-13Y  [P1-13Y]
C1  100u/16V  CPOL-EUUD-6,3X8,8  [UD-6,3X5,8_NICHICON]
C1P  100n  C-EUC1206  [C1206]
C2P  100n  C-EUC1206  [C1206]
C3P  100n  C-EUC1206  [C1206]
C6N  100n  C-EUC1206  [C1206]
C6P  100n  C-EUC1206  [C1206]
C7N  100n  C-EUC1206  [C1206]
C7P  100n  C-EUC1206  [C1206]
C8  100n  C-EUC1206  [C1206]
C8N  100n  C-EUC1206  [C1206]
C8P  100n  C-EUC1206  [C1206]
C9N  100n  C-EUC1206  [C1206]
C9N1  10u/25V  CPOL-EUUD-4X5,8  [UD-4X5,8_NICHICON]
C9P  100n  C-EUC1206  [C1206]
C9P1  10u/25V  CPOL-EUUD-4X5,8  [UD-4X5,8_NICHICON]
C10N  100n  C-EUC1206  [C1206]
C10P  100n  C-EUC1206  [C1206]
C11N  100n  C-EUC1206  [C1206]
C11P  100n  C-EUC1206  [C1206]
C12N  100n  C-EUC1206  [C1206]
C12P  100n  C-EUC1206  [C1206]
C13N  100n  C-EUC1206  [C1206]
C13P  100n  C-EUC1206  [C1206]
C14  100n  C-EUC1206  [C1206]
C14N  100n  C-EUC1206  [C1206]
C14P  100n  C-EUC1206  [C1206]
C15  100u/16V  CPOL-EUUD-6,3X8,8  [UD-6,3X5,8_NICHICON]
C15N  100n  C-EUC1206  [C1206]
C15P  100n  C-EUC1206  [C1206]
C16  100n  C-EUC1206  [C1206]
C16N  100n  C-EUC1206  [C1206]
C16P  100n  C-EUC1206  [C1206]
C17N  100n  C-EUC1206  [C1206]
C17P  100n  C-EUC1206  [C1206]
C18  100u/16V  CPOL-EUUD-6,3X8,8  [UD-6,3X5,8_NICHICON]
C18N  100n  C-EUC1206  [C1206]
C18P  100n  C-EUC1206  [C1206]
C19N  100n  C-EUC1206  [C1206]
C19P  100n  C-EUC1206  [C1206]
C21N  100n  C-EUC1206  [C1206]
C21P  100n  C-EUC1206  [C1206]
C23N  100n  C-EUC1206  [C1206]
C23P  100n  C-EUC1206  [C1206]
C24N  100n  C-EUC1206  [C1206]
C24P  100n  C-EUC1206  [C1206]
C29  100n  C-EUC1206  [C1206]
C30  100n  C-EUC1206  [C1206]
C35  100u/16V  CPOL-EUUD-6,3X8,8  [UD-6,3X5,8_NICHICON]
C36  100u/16V  CPOL-EUUD-6,3X8,8  [UD-6,3X5,8_NICHICON]
C37  1u/50V  CPOL-EUUD-4X5,8  [UD-4X5,8_NICHICON]
C38  1u/50V  CPOL-EUUD-4X5,8  [UD-4X5,8_NICHICON]
GND  TPPAD1-13Y  [P1-13Y]
IC120  7812TV  [TO220V]
IC130  7805TV  [TO220V]
L5  10u  L-USL3216C  [L3216C]
L7  10u  L-USL3216C  [L3216C]

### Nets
+5V: C1.+ C1P.1 C2P.1 C3P.1 C8.1 IC1.16(VCC) IC2.16(VCC) IC3.16(VCC) IC130.3(VO) ; also sheet 3
+12V: C15.+ C16.1 IC120.3(VO) IC130.1(VI) ; also sheet 3
+15V: +15V.TP C6P.1 C7P.1 C8P.1 C10P.1 C11P.1 C12P.1 C13P.1 C14.1 C14P.1 C15P.1 C16P.1 C17P.1 C18.+ C18P.1 C19P.1 C21P.1 C23P.1 C24P.1 C29.1 C35.+ C37.+ IC120.1(VI) L7.1 ; also sheet 1,2,5
-15V: -15V.TP C6N.2 C7N.2 C8N.2 C10N.2 C11N.2 C12N.2 C13N.2 C14N.2 C15N.2 C16N.2 C17N.2 C18N.2 C19N.2 C21N.2 C23N.2 C24N.2 C30.2 C36.- C38.- L5.1 ; also sheet 1,2,5
GND: C1.- C1P.2 C2P.2 C3P.2 C6N.1 C6P.2 C7N.1 C7P.2 C8.2 C8N.1 C8P.2 C9N1.+ C9N.1 C9P1.- C9P.2 C10N.1 C10P.2 C11N.1 C11P.2 C12N.1 C12P.2 C13N.1 C13P.2 C14.2 C14N.1 C14P.2 C15.- C15N.1 C15P.2 C16.2 C16N.1 C16P.2 C17N.1 C17P.2 C18.- C18N.1 C18P.2 C19N.1 C19P.2 C21N.1 C21P.2 C23N.1 C23P.2 C24N.1 C24P.2 C29.2 C30.1 C35.- C36.+ C37.- C38.+ GND.TP IC1.8(GND) IC2.8(GND) IC3.8(GND) IC120.2(GND) IC130.2(GND) ; also sheet 1,2,3,5
IC9+15V: C9P1.+ C9P.1 L7.2 ; also sheet 1
IC9-15V: C9N1.- C9N.2 L5.2 ; also sheet 1

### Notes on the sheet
- PCB2 Sheet 4: Power-Supply

## Sheet 5 of 5: Analog Interface
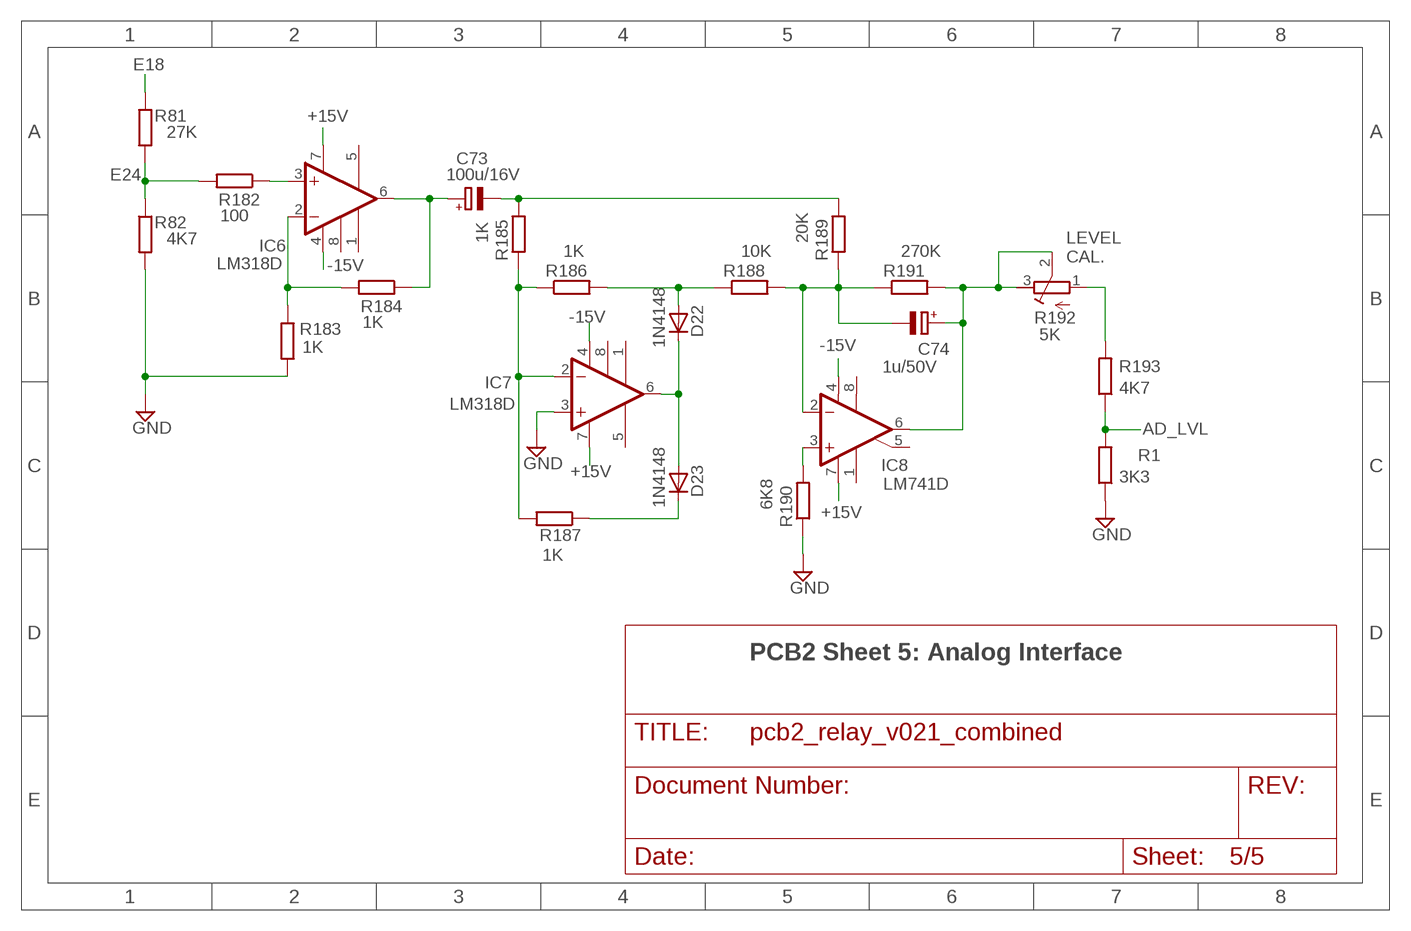
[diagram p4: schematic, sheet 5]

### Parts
C73  100u/16V  CPOL-EUUD-6,3X8,8  [UD-6,3X5,8_NICHICON]
C74  1u/50V  CPOL-EUUD-4X5,8  [UD-4X5,8_NICHICON]
D22  1N4148  D-SOD-80  [SOD80]
D23  1N4148  D-SOD-80  [SOD80]
IC6  LM318D  [SOIC8]
IC7  LM318D  [SOIC8]
IC8  LM741D  [SO08]
R1  3K3  R-EU_R1206  [R1206]
R81  27K  R-EU_R1206  [R1206]
R82  4K7  R-EU_R1206  [R1206]
R182  100  R-EU_R1206  [R1206]
R183  1K  R-EU_R1206  [R1206]
R184  1K  R-EU_R1206  [R1206]
R185  1K  R-EU_R1206  [R1206]
R186  1K  R-EU_R1206  [R1206]
R187  1K  R-EU_R1206  [R1206]
R188  10K  R-EU_R1206  [R1206]
R189  20K  R-EU_R1206  [R1206]
R190  6K8  R-EU_R1206  [R1206]
R191  270K  R-EU_R1206  [R1206]
R192  5K  R-TRIMM3296W  [RTRIM3296W]
R193  4K7  R-EU_R1206  [R1206]

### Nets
+15V: IC6.7(V+) IC7.7(V+) IC8.7(V+) ; also sheet 1,2,4
-15V: IC6.4(V-) IC7.4(V-) IC8.4(V-) ; also sheet 1,2,4
AD_LVL: R1.2 R193.1 ; also sheet 3
E18: R81.1 ; also sheet 1,2,3
E24: R81.2 R82.1 R182.2
GND: IC7.3(+IN) R1.1 R82.2 R183.2 R190.1 ; also sheet 1,2,3,4
N$1: IC6.3(+IN) R182.1
N$2: IC8.3(+IN) R190.2
N$10: IC6.2(-IN) R183.1 R184.2
N$11: C73.+ IC6.6(OUT) R184.1
N$13: R192.1(A) R193.2
N$14: IC7.2(-IN) R185.1 R186.1 R187.2
N$15: D23.1(C) R187.1
N$16: D22.1(C) D23.2(A) IC7.6(OUT)
N$18: D22.2(A) R186.2 R188.1
N$19: C74.- IC8.2(-IN) R188.2 R189.1 R191.1
N$20: C74.+ IC8.6(OUT) R191.2 R192.2(S) R192.3(E)
N$23: C73.- R185.2 R189.2
Unconnected: IC6.1(BAL1) IC6.5(BAL2) IC6.8(COMP) IC7.1(BAL1) IC7.5(BAL2) IC7.8(COMP) IC8.1(ON1) IC8.5(ON2) IC8.8(OPT)

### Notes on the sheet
- LEVEL
  CAL.
- PCB2 Sheet 5: Analog Interface

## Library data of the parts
+15V -15V E15-E23 E28-E32 GND GNDI INPUT = testpad:TP: Test pad
C1 C9N1 C9P1 C15 C18 C23 C35-C38 C41-C50 C73 C74 = rcl:CPOL-EU: POLARIZED CAPACITOR, European symbol; SPICEPREFIX: C
C1P C2P C3P C6N C6P C7N C7P C8 C8N C8P C9N C9P C10N C10P C11N C11P C12N C12P C13N C13P C14 C14N C14P C15N C15P C16 C16N C16P C17N C17P C18N C18P C19N C19P C21N C21P C22 C23N C23P C24 C24N C24P C25-C30 C51 C75 C210 C211 C222 COQ1-COQ4 CPR1-CPR4 = rcl:C-EU: CAPACITOR, European symbol; SPICEPREFIX: C
C3-C5 = rcl:C-TRIMM: Trimm capacitor; SPICEPREFIX: C
CON1 CON2 = Wurth_Elektronik_Electromechanic_Wire_to_Board_Connectors_rev16a:61200821621: WR-BHD 2.54mm Male Box Header, 8 Pins=>Code : Con_WTB_BHD_2.54_Male_THT_WS_61200821621 Details see: http://katalog.we-online.de/en/em/612_0xx_216_21 Created 2014-06-04, Karrer Zheng 2014 (C) Würth Elektronik
D4-D11 D22 D23 = semicon-smd-ipc:D-: DIODE
DS1-DS13 DS15-DS24 = diode:DIODE-: DIODE
IC1-IC3 = 74xx-eu:74*595: 8-bit SHIFT REGISTER, output latch
IC6 IC7 = linear:LM*18: FAST GENERAL-PURPOSE OPERATIONAL AMPLIFIER Sourde: http://focus.ti.com/lit/ds/slos063b/slos063b.pdf
IC8 = linear:*741: OP AMP
IC9-IC17 = linear:NE5534: LOW-NOISE OPERATIONAL AMPLIFIER Source: http://focus.ti.com/lit/ds/symlink/ne5534.pdf
IC18 IC19 IC21 IC23 = linear:LM318: OP AMP
IC20 IC22 = emile:MC1496
IC24 = linear:LF356: OP AMP
IC120 IC130 = linear:78*: Positive VOLTAGE REGULATOR Source: http://cache.national.com/ds/LM/LM78L05.pdf http://www.fairchildsemi.com/ds/LM/LM7805.pdf
K1-K13 K15-K24 = relay:G6K: Low Signal Relay oeiwcsnts1.omron.com/.. D20G6K0100.pdf; MF: OMRON COMPONENTS USA; MPN: G6K-2F-Y DC3; OC_FARNELL: 1690316; OC_NEWARK: 89C6451
L1-L4 = dp_devices:FERRITE: Ferrite bead in various packages
L5 L7 = rcl:L-US: INDUCTOR, American symbol; SPICEPREFIX: L
Q5 Q6 = transistor-small-signal:2N5638: N-CHANNEL FET
QS1-QS13 QS15-QS24 = semicon-smd-ipc:NPN-TRANSISTOR_: NPN TRANSISTOR
R1 R44-R58 R60 R61 R63-R86 R88-R124 R182-R191 R193 R213 R214 RG1-RG11 RH1-RH11 ROQ4 RPR4 = rcl:R-EU_: RESISTOR, European symbol; SPICEPREFIX: R
R59 R62 R192 = rcl:R-TRIMM: Trimm resistor; SPICEMODEL: X; SPICEPREFIXL: POT
RS1-RS13 RS15-RS24 = rcl:R-EU_: RESISTOR, European symbol

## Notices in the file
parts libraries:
Wurth_Elektronik_Electromechanic_Wire_to: Copyright: Würth Elektronik
